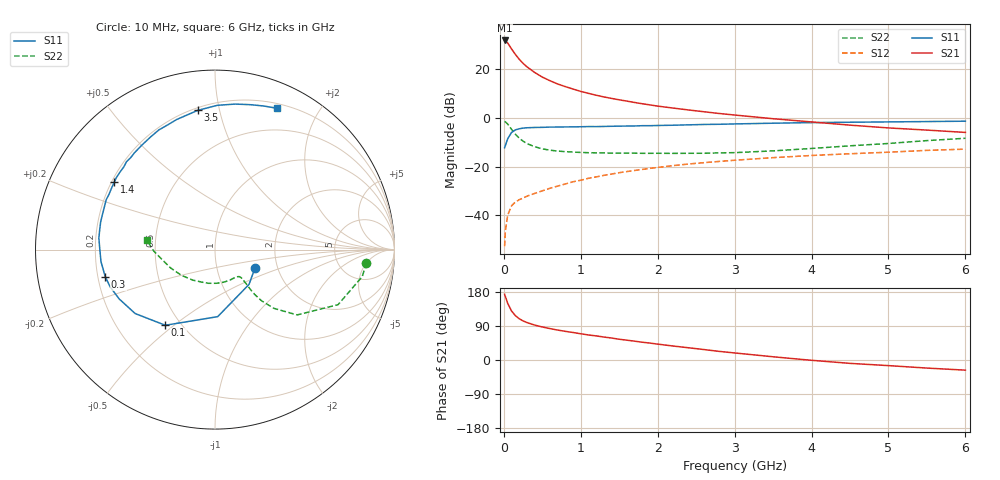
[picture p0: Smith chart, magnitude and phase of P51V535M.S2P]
! SIEMENS Small Signal Semiconductors
! BFP183
! Si NPN RF Bipolar Junction Transistor in SOT143
! VCE = 1.5 V  IC = 35 mA
! Common Emitter S-Parameters:  March  1996
# GHz  S  MA  R  50
!  f  S11  S21  S12  S22
! GHz  MAG  ANG  MAG  ANG  MAG  ANG  MAG  ANG
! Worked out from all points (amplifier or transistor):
!   36 points, 10 MHz to 6 GHz, reference 50 ohm
!   highest |S21| = 31.9 dB at 10 MHz (marker M1)
!   |S21| within 3 dB of that: start of sweep to 89.93 MHz
!   unconditionally stable (mu >= 1): start of sweep to 14.94 MHz; 338.8 MHz to end of sweep
!   at 250 MHz: K = 0.85, MSG = 27.7 dB, |S12| = -33.0 dB
!   at 1.4 GHz: K = 1.45, MAG = 11.6 dB, |S12| = -23.1 dB
!   at 6 GHz: K = 1.13, MAG = 1.3 dB, |S12| = -12.8 dB
!   S11 on the Smith chart (normalised r, x): 10 MHz: 1.53, -0.33; 100 MHz: 0.41, -0.47; 300 MHz: 0.23, -0.12; 1.4 GHz: 0.21, +0.29; 3.5 GHz: 0.22, +0.86; 6 GHz: 0.25, +1.50
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0.01  0.245 -24.3  39.49 173.5  0.0023 75.2  0.8471 -5.0
0.02  0.2712 -45.6  39.14 167.2  0.0048 70.7  0.8339 -10.4
0.05  0.3739 -87.7  35 149.6  0.01 68.0  0.7512 -24.1
0.1  0.5044 -123.3  26.41 129.4  0.0156 51.6  0.5845 -38.5
0.15  0.5698 -141.3  20.38 117.1  0.0187 48.0  0.4638 -44.9
0.2  0.6003 -152.7  16.22 108.9  0.0208 46.7  0.3857 -47.7
0.25  0.6198 -160.3  13.34 103.1  0.0225 46.7  0.334 -48.5
0.3  0.6298 -166.1  11.34 98.9  0.0246 48.4  0.2978 -48.4
0.4  0.6388 -174.0  8.676 92.2  0.028 51.1  0.2565 -47.6
0.5  0.6422 179.5  6.95 87.1  0.0317 52.4  0.2319 -47.2
0.6  0.6503 174.3  5.854 82.9  0.0358 55.0  0.2174 -47.0
0.7  0.6519 170.2  5.006 79.0  0.0397 56.6  0.2086 -47.3
0.8  0.6555 166.4  4.426 75.6  0.0439 57.2  0.2029 -48.0
1.1  0.6668 155.4  3.218 66.1  0.0574 58.1  0.1931 -52.3
1.4  0.6757 146.3  2.534 58.0  0.0702 57.4  0.1895 -58.7
1.8  0.6948 135.2  1.966 46.9  0.0873 54.9  0.1876 -68.9
2.2  0.7104 125.0  1.602 36.9  0.1046 51.4  0.1871 -80.7
2.8  0.7429 110.9  1.239 22.7  0.1277 45.2  0.1914 -101.4
3.5  0.7816 97.1  0.967 8.5  0.1528 38.6  0.2106 -126.2
4.5  0.8186 82.1  0.713 -8.9  0.1838 28.6  0.2675 -157.5
5.5  0.8453 71.1  0.564 -21.3  0.2158 19.7  0.3427 -178.9
6  0.8598 66.3  0.505 -26.8  0.2287 14.6  0.3829 172.2
